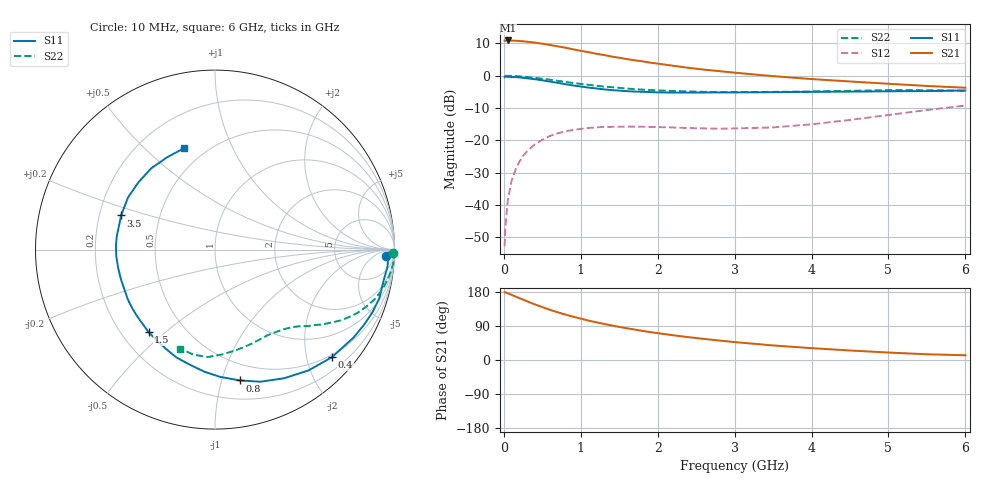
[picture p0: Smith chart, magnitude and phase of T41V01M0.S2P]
! Infineon Technologies  Discrete & RF Semiconductors
! BFR182T
! Si NPN RF Bipolar Junction Transistor in SC75
! VCE = 1 V  IC = 1 mA
! Common Emitter S-Parameters:  October  1999
# GHz  S  MA  R  50
!  f  S11  S21  S12  S22
! GHz  MAG  ANG  MAG  ANG  MAG  ANG  MAG  ANG
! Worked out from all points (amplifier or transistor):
!   36 points, 10 MHz to 6 GHz, reference 50 ohm
!   highest |S21| = 10.9 dB at 50 MHz (marker M1)
!   |S21| within 3 dB of that: start of sweep to 954.9 MHz
!   unconditionally stable (mu >= 1): 2.306 GHz to 4.894 GHz
!   at 250 MHz: K = 0.10, MSG = 17.8 dB, |S12| = -24.9 dB
!   at 1.4 GHz: K = 0.61, MSG = 10.9 dB, |S12| = -15.8 dB
!   at 6 GHz: K = 0.92, MSG = 2.8 dB, |S12| = -9.2 dB
!   S11 on the Smith chart (normalised r, x): 10 MHz: 26, -20; 400 MHz: 0.45, -2.49; 800 MHz: 0.35, -1.14; 1.5 GHz: 0.31, -0.44; 3.5 GHz: 0.29, +0.16; 6 GHz: 0.38, +0.67
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0.01  0.9524 -2.1  3.494 178.7  0.0023 85.0  0.9912 -1.2
0.02  0.9673 -0.9  3.501 178.7  0.0045 99.4  0.9941 -0.9
0.05  0.9659 -5.6  3.524 175.9  0.0116 91.9  0.996 -2.3
0.1  0.9549 -10.5  3.496 172.1  0.0234 83.7  0.9951 -4.6
0.15  0.9548 -16.6  3.49 167.6  0.0347 80.4  0.9872 -6.9
0.25  0.93 -26.8  3.421 159.3  0.0572 74.1  0.9692 -11.2
0.4  0.8854 -42.6  3.269 147.0  0.0864 65.3  0.9314 -17.3
0.5  0.8515 -52.2  3.14 139.6  0.102 59.7  0.9003 -20.7
0.6  0.8139 -61.7  2.997 132.4  0.1169 54.9  0.8693 -23.9
0.7  0.7785 -71.0  2.856 126.0  0.1288 50.6  0.8362 -26.7
0.8  0.7419 -79.3  2.722 119.9  0.138 46.6  0.8049 -29.3
0.9  0.7093 -87.8  2.571 114.3  0.1447 42.9  0.7751 -31.4
1.1  0.6554 -102.7  2.322 103.9  0.1558 37.2  0.7247 -35.2
1.3  0.6166 -116.4  2.1 95.3  0.1618 32.7  0.6822 -38.4
1.5  0.59 -128.9  1.905 87.3  0.1627 29.8  0.6505 -41.0
1.8  0.5641 -145.6  1.674 76.8  0.1627 26.5  0.611 -45.0
2.2  0.5495 -162.3  1.431 65.3  0.1583 25.9  0.5826 -50.1
2.8  0.5524 178.1  1.18 51.4  0.1518 29.7  0.5595 -59.0
3.5  0.5565 160.0  0.987 38.4  0.1587 40.0  0.5632 -69.4
4.5  0.5679 139.0  0.816 25.1  0.2074 52.1  0.5848 -85.5
5.5  0.5795 117.2  0.696 15.1  0.295 54.0  0.5974 -101.6
6  0.5915 106.7  0.653 12.5  0.3457 51.5  0.5852 -109.3
